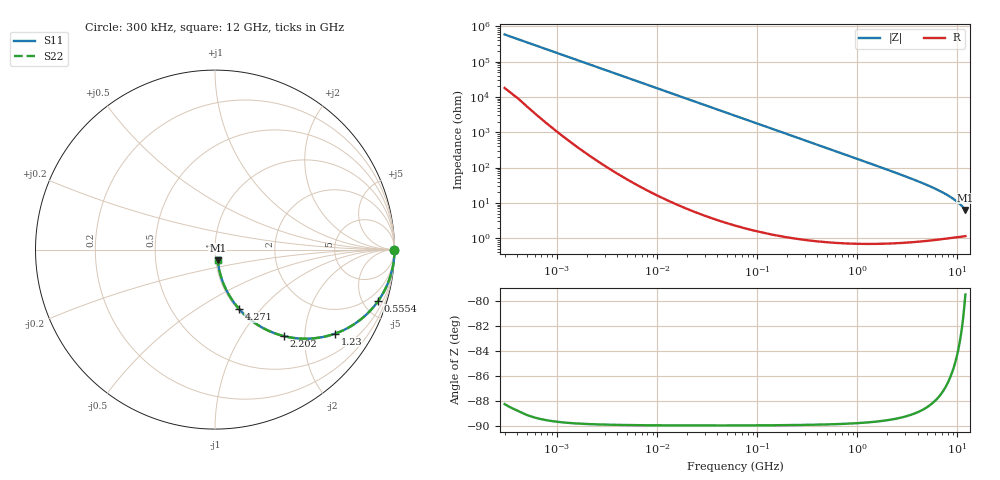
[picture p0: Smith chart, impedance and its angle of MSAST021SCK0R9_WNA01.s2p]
! MSAST021SCK0R9_WNA01  S-PARAMETER MODEL  ( General Type )
! Model Generated by TAIYO YUDEN Corporation (http://www.ty-top.com)
! Version 2.0
! TAIYO YUDEN Control No. 181101
! Copyright(c) 2015 TAIYO YUDEN CO.,LTD. All Rights Reserved.
! Product Description (link to TY-COMPAS)
! https://ds.yuden.co.jp/TYCOMPAS/or/detail?pn=MSAST021SCK0R9BWNA01&u=M
! Products Name : Multilayer Ceramic Capacitors
! Characteristics :
!  Capacitance : 0.9 pF , Rated Voltage : 25V , TCC : CK / C0K
!  Case Size : 0.25 x 0.125 / 0.0098 x 0.0049 [mm/inch] , Thickness : 0.125 / 0.0049 [mm/inch]
!  (Conditions: Temperature = 25 degC , DC Bias Current/Voltage = 0A / 0V)
! External Node Assignments :
!  1  o---| |---o  2
! GND o---------o GND
! Frequency Range : 0.3MHz  -  12000MHz  [ 401 STEP ]
# MHz S RI R 50
! Freq[MHz].  S11 Real  S11 Imag  S21 Real  S21 Imag  S12 Real  S12 Imag  S22 Real  S22 Imag
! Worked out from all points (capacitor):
!   401 points, 300 kHz to 12 GHz, reference 50 ohm
!   read as one part in series: C = 900 fF near 316.3 kHz
!   lowest |Z| = 6.29 ohm at 12 GHz (marker M1)
!   S11 on the Smith chart (normalised r, x): 300 kHz: open; 555.4 MHz: 1.01, -6.36; 1.23 GHz: 1.01, -2.86; 2.202 GHz: 1.01, -1.57; 4.271 GHz: 1.02, -0.77; 12 GHz: 1.02, -0.12
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0.3  1 -0.000169  5.2e-06 0.000169  5.2e-06 0.000169  1 -0.000169
0.316324  1 -0.000179  5.14e-06 0.000179  5.14e-06 0.000179  1 -0.000179
1.769972  1 -0.001  4.1e-06 0.001  4.1e-06 0.001  1 -0.001
10.44266  1 -0.0059  4.02e-05 0.0059  4.02e-05 0.0059  1 -0.0059
60  0.9988 -0.0339  0.00118 0.0339  0.00118 0.0339  0.9988 -0.0339
159.8975  0.9918 -0.0897  0.00821 0.0897  0.00821 0.0897  0.9918 -0.0897
244.3004  0.9811 -0.1355  0.0189 0.1355  0.0189 0.1355  0.9811 -0.1355
353.9943  0.9611 -0.1924  0.0389 0.1924  0.0389 0.1924  0.9611 -0.1924
555.3718  0.9095 -0.2858  0.0905 0.2858  0.0905 0.2858  0.9095 -0.2858
826.3444  0.8192 -0.3832  0.1808 0.3832  0.1808 0.3832  0.8192 -0.3832
994.7115  0.7573 -0.4267  0.2427 0.4267  0.2427 0.4267  0.7573 -0.4267
1229.528  0.6707 -0.4676  0.3293 0.4676  0.3293 0.4676  0.6707 -0.4676
1602.47  0.5437 -0.4949  0.4563 0.4949  0.4563 0.4949  0.5437 -0.4949
2088.533  0.4097 -0.4876  0.5903 0.4876  0.5903 0.4876  0.4097 -0.4876
2202.174  0.3837 -0.4818  0.6163 0.4818  0.6163 0.4818  0.3837 -0.4818
3107.553  0.2333 -0.4162  0.7667 0.4162  0.7667 0.4162  0.2333 -0.4162
4270.516  0.1335 -0.3298  0.8665 0.3298  0.8665 0.3298  0.1335 -0.3298
6026.253  0.0664 -0.2318  0.9336 0.2318  0.9336 0.2318  0.0664 -0.2318
7854.144  0.0367 -0.1614  0.9633 0.1614  0.9633 0.1614  0.0367 -0.1614
9708.23  0.0227 -0.1092  0.9773 0.1092  0.9773 0.1092  0.0227 -0.1092
11380.75  0.0164 -0.0722  0.9836 0.0722  0.9836 0.0722  0.0164 -0.0722
12000  0.015 -0.0602  0.985 0.0602  0.985 0.0602  0.015 -0.0602
